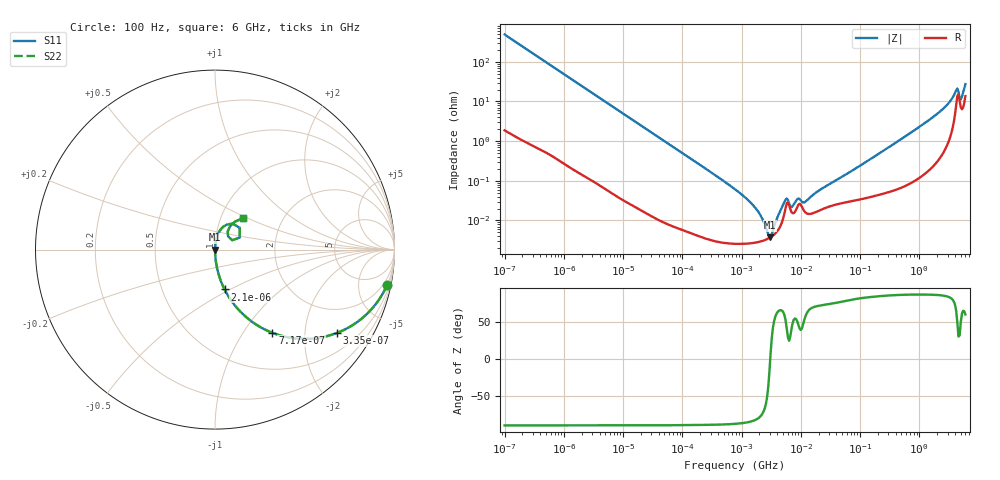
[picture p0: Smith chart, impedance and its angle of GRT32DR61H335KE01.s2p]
!Murata Part Number: GRT32DR61H335KE01
!These Parameters are Measured in Series Mode Connection
!Data Generated on Jun 19, 2026
!  o--ll--o
!Port1  Port2
!  o------o
!Operation Temp=25[degC], DC Bias Voltage=0[V]
!Freq. Start=100[Hz] Stop=6[GHz] 401[Steps]
# Hz S RI R 50
!Freq.(Hz) S11(Real) S11(Imag) S21(Real) S21(Imag) S12(Real) S12(Imag) S22(Real) S22(Imag)
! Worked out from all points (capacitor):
!   401 points, 100 Hz to 6 GHz, reference 50 ohm
!   read as one part in series: C = 3.26 uF near 109 Hz
!   lowest |Z| = 3.77 mohm at 2.968 MHz (marker M1)
!   series resonance near 3.048 MHz, so ESL is about 840 pH
!   S11 on the Smith chart (normalised r, x): 100 Hz: 1.04, -9.76; 335 Hz: 1.01, -2.92; 717 Hz: 1.01, -1.37; 2.1 kHz: 1.00, -0.47; 6 GHz: 1.27, +0.47
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100  0.959 -0.1964  0.041 0.1964  0.041 0.1964  0.959 -0.1964
335  0.6801 -0.464  0.3199 0.464  0.3199 0.464  0.6801 -0.464
717  0.3198 -0.4637  0.6802 0.4637  0.6802 0.4637  0.3198 -0.4637
2008  0.0579 -0.2307  0.9421 0.2307  0.9421 0.2307  0.0579 -0.2307
2100  0.0533 -0.2217  0.9467 0.2217  0.9467 0.2217  0.0533 -0.2217
6728  0.00584 -0.0731  0.9942 0.0731  0.9942 0.0731  0.00584 -0.0731
40335  0.000254 -0.0123  0.9997 0.0123  0.9997 0.0123  0.000254 -0.0123
774597  2.61e-05 -0.000611  1 0.000611  1 0.000611  2.61e-05 -0.000611
1449809  2.67e-05 -0.000272  1 0.000272  1 0.000272  2.67e-05 -0.000272
2372521  3.13e-05 -8.67e-05  1 8.67e-05  1 8.67e-05  3.13e-05 -8.67e-05
2967816  3.65e-05 -9.3e-06  1 9.3e-06  1 9.3e-06  3.65e-05 -9.3e-06
3882480  5.06e-05 9.14e-05  0.9999 -9.14e-05  0.9999 -9.14e-05  5.06e-05 9.14e-05
5554849  0.000209 0.000263  0.9998 -0.000263  0.9998 -0.000263  0.000209 0.000263
7266822  0.000152 0.000171  0.9998 -0.000171  0.9998 -0.000171  0.000152 0.000171
8692127  0.000216 0.000267  0.9998 -0.000267  0.9998 -0.000267  0.000216 0.000267
1.137099e7  0.000175 0.000223  0.9998 -0.000223  0.9998 -0.000223  0.000175 0.000223
1.555665e7  0.00015 0.000397  0.9998 -0.000397  0.9998 -0.000397  0.00015 0.000397
3.124326e8  0.000574 0.00714  0.9994 -0.00714  0.9994 -0.00714  0.000574 0.00714
2.048624e9  0.0056 0.0495  0.9944 -0.0495  0.9944 -0.0495  0.0056 0.0495
4.009986e9  0.0663 0.1398  0.9337 -0.1398  0.9337 -0.1398  0.0663 0.1398
5.245841e9  0.0707 0.1014  0.9293 -0.1014  0.9293 -0.1014  0.0707 0.1014
6e9  0.1569 0.1761  0.8431 -0.1761  0.8431 -0.1761  0.1569 0.1761
